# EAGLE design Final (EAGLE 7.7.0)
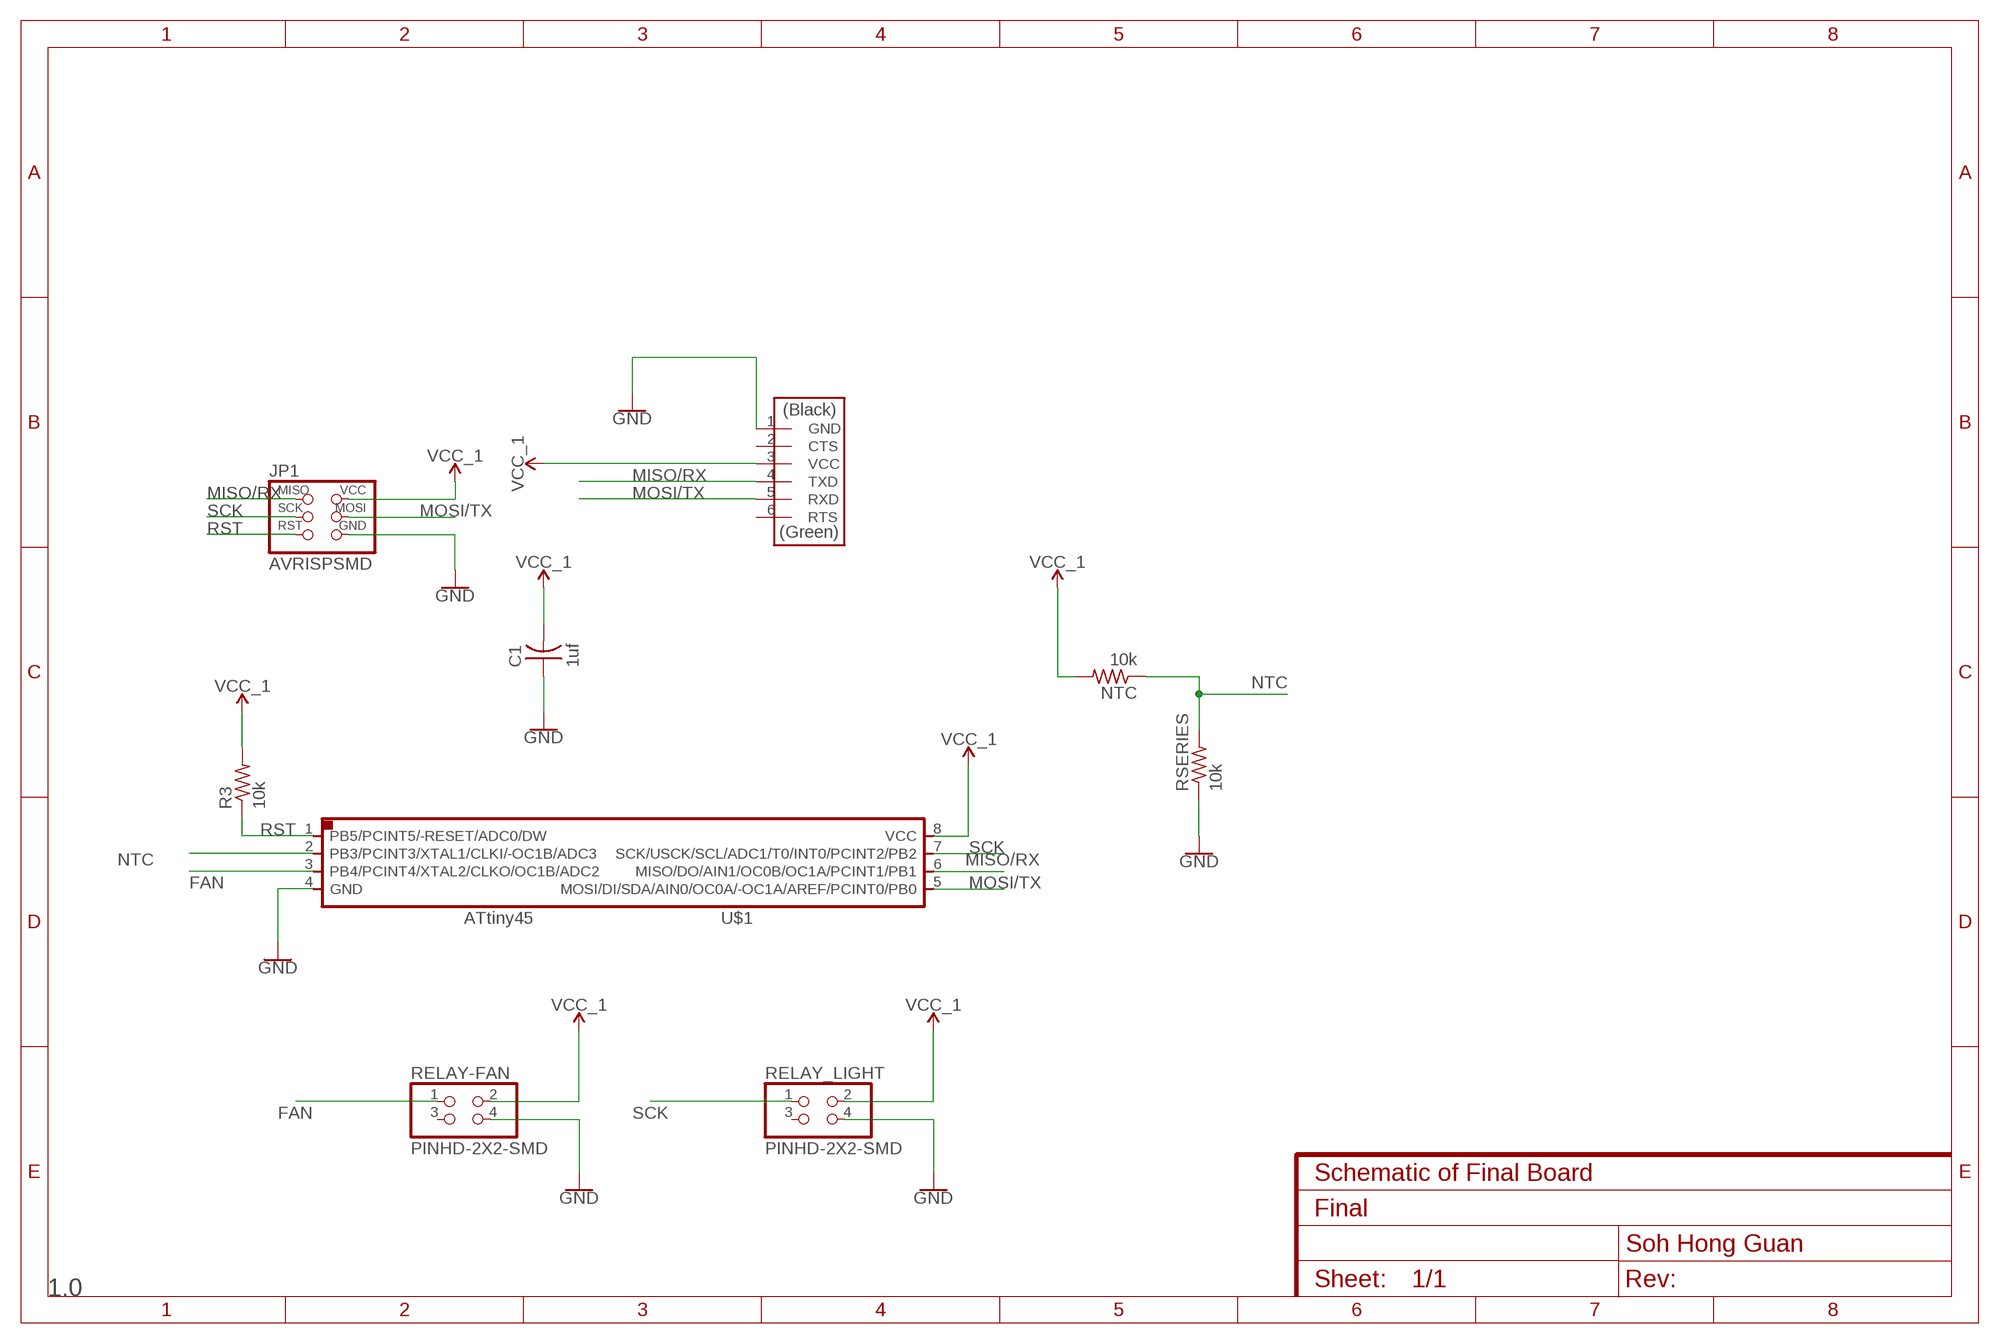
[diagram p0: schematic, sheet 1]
FRAME1 (FRAME-A4L): CNAME: Schematic of Final Board; CREVISION: 1.0; DESIGNER: Soh Hong Guan

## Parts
C1  1uf  CAP-US1206  [C1206]
JP1  AVRISPSMD  [2X03SMD]
NTC  10k  RES-US1206  [R1206]
R3  10k  RES-US1206  [R1206]
RELAY-FAN  PINHD-2X2-SMD  [2X02SMD]
RELAY_LIGHT  PINHD-2X2-SMD  [2X02SMD]
RSERIES  10k  RES-US1206  [R1206]
U$1  ATTINY45SI  [SOIC8]
U$3  FTDI-SMD-HEADER  [1X06SMD]

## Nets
FAN: RELAY-FAN.1 U$1.3(PB4/PCINT4/XTAL2/CLKO/OC1B/ADC2)
GND: C1.1 JP1.6(GND) RELAY-FAN.4 RELAY_LIGHT.4 RSERIES.1 U$1.4(GND) U$3.1(GND)
MISO/RX: JP1.1(MISO) U$1.6(MISO/DO/AIN1/OC0B/OC1A/PCINT1/PB1) U$3.4(TXD)
MOSI/TX: JP1.4(MOSI) U$1.5(MOSI/DI/SDA/AIN0/OC0A/-OC1A/AREF/PCINT0/PB0) U$3.5(RXD)
NTC: NTC.1 RSERIES.2 U$1.2(PB3/PCINT3/XTAL1/CLKI/-OC1B/ADC3)
RST: JP1.5(RST) R3.1 U$1.1(PB5/PCINT5/-RESET/ADC0/DW)
SCK: JP1.3(SCK) RELAY_LIGHT.1 U$1.7(SCK/USCK/SCL/ADC1/T0/INT0/PCINT2/PB2)
VCC_1: C1.2 JP1.2(VCC) NTC.2 R3.2 RELAY-FAN.2 RELAY_LIGHT.2 U$1.8(VCC) U$3.3(VCC)
Unconnected: RELAY-FAN.3 RELAY_LIGHT.3 U$3.2(CTS) U$3.6(RTS)

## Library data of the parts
C1 = fab:CAP-US
JP1 = fab:AVRISP
NTC R3 RSERIES = fab:RES-US: Resistor (US Symbol)
RELAY-FAN RELAY_LIGHT = fab:PINHD-2X2-SMD
U$1 = fab:ATTINY45
U$3 = fab:FTDI-SMD-HEADER

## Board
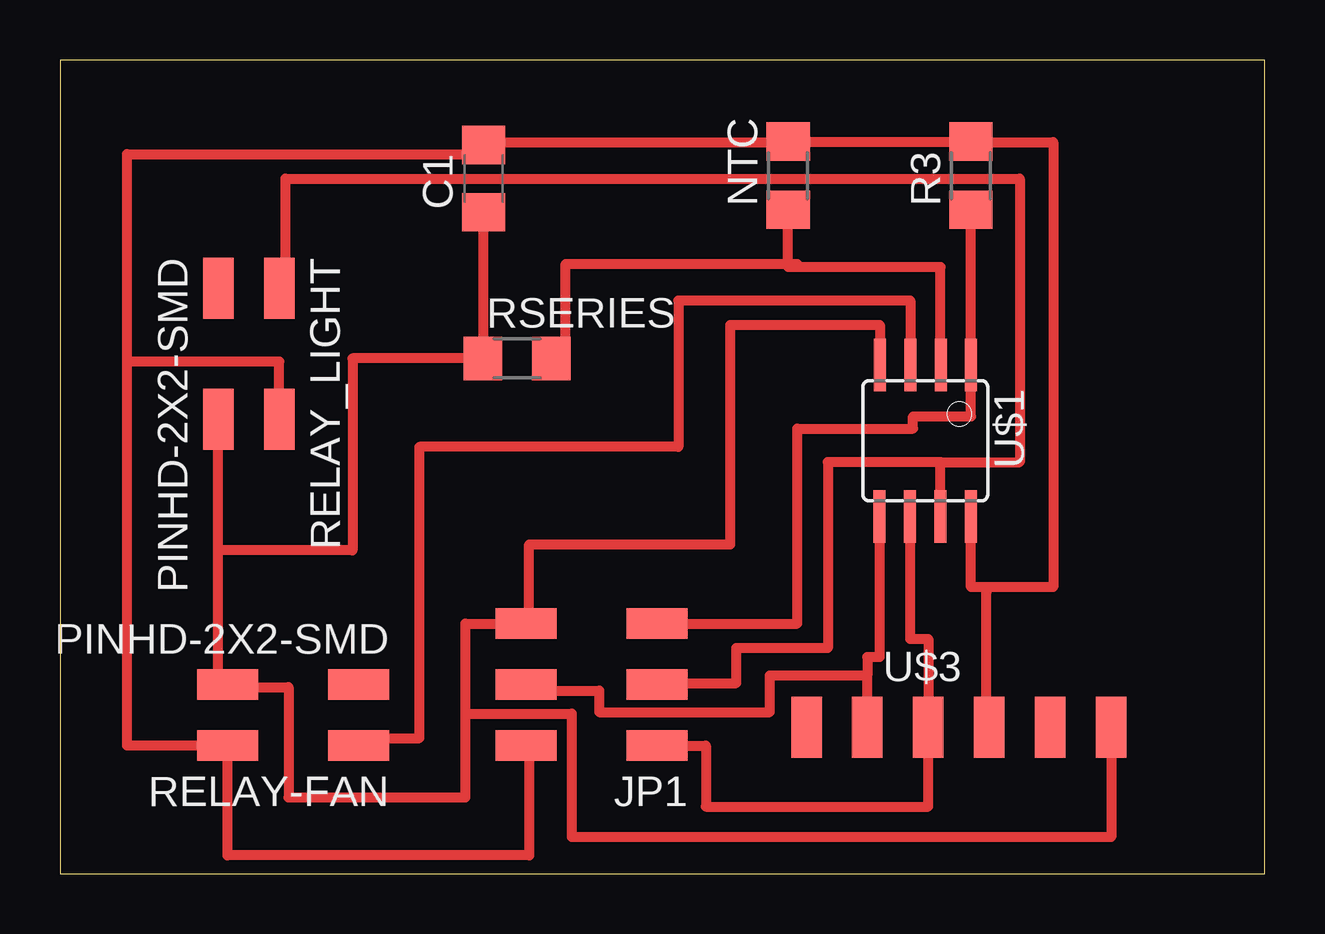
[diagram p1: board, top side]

Size 50.22 x 33.9 mm. Coordinates in mm from the lower left corner, seen from the top.
Outline: 0,0 50.22,0 50.22,33.9 0,33.9 0,0
Copper layers (1*16): Top 0.035mm / dielectric 1.5mm / Bottom 0.035mm
Design rules "default *": minimum track width 16mil, minimum drill 24mil, track to track 12mil, track to pad 12mil, pad to pad 12mil, via to via 8mil, smd to smd 12mil, copper to edge 40mil, drill to drill 8mil, minimum pad ring 10mil, minimum via ring 8mil, stop-mask expansion 4mil, vias tented up to drill 0mil, thermal gap 10mil

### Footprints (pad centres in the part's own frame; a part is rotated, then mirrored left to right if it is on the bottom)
C1206 = smd 1.6 x 1.8: 1 -1.4,0; 2 1.4,0
2X03SMD = smd 2.54 x 1.27: 1 -2.54,2.54; 2 2.92,2.54; 3 -2.54,0; 4 2.92,0; 5 -2.54,-2.54; 6 2.92,-2.54
R1206 = smd 1.6 x 1.803: 1 -1.422,0; 2 1.422,0
2X02SMD = smd 2.54 x 1.27: 1 -2.54,1.27; 2 2.92,1.27; 3 -2.54,-1.27; 4 2.92,-1.27
SOIC8 = smd 0.5 x 2.2: 1 -1.905,-3.154; 2 -0.645,-3.154; 3 0.625,-3.154; 4 1.895,-3.154; 5 1.905,3.154; 6 0.635,3.154; 7 -0.635,3.154; 8 -1.905,3.154
1X06SMD = smd 2.54 x 1.27: 1 0,6.35; 2 0,3.81; 3 0,1.27; 4 0,-1.27; 5 0,-3.81; 6 0,-6.35

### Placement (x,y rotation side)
C1  17.65,28.96 90 top
JP1  22.35,7.87 180 top
NTC  30.35,29.08 90 top
R3  37.97,29.08 90 top
RELAY-FAN  9.91,6.6 180 top
RELAY_LIGHT  7.87,21.84 270 top
RSERIES  19.05,21.46 0 top
U$1  36.07,18.03 180 top
U$3  37.47,6.1 270 top

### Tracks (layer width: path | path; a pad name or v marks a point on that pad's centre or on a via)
FAN
  Top 0.406: RELAY-FAN.1 12.45,5.64 14.99,5.64 14.99,17.78 25.78,17.78 25.78,23.88 35.44,23.88 U$1.3
GND
  Top 0.406: 34.14,20.93 U$1.4 34.17,22.86 27.94,22.86 27.94,13.72 19.56,13.72 19.56,10.62 JP1.6 | 19.2,10.62 JP1.6 | 6.6,19.15 6.76,19.15 RELAY_LIGHT.4 6.6,13.46 | JP1.6 16.89,10.41 16.89,6.67 | C1.1 17.63,27.56 RSERIES.1 12.19,21.46 12.19,13.46 6.6,13.46 | 6.6,13.46 6.6,8.13 7.11,8.13 RELAY-FAN.4 7.11,7.77 9.53,7.77 9.53,3.17 16.89,3.17 16.89,6.67 | 16.89,6.67 21.34,6.67 21.34,1.52 43.81,1.52 U$3.1
MISO/RX
  Top 0.406: JP1.1 26.92,5.33 26.92,2.79 36.2,2.79 U$3.4 36.2,9.78 35.43,9.78 U$1.6
MOSI/TX
  Top 0.406: U$3.5 33.66,8.26 | JP1.4 19.68,7.62 22.48,7.62 22.48,6.73 29.59,6.73 29.59,8.26 33.66,8.26 | U$1.5 34.16,9.02 33.66,9.02 33.66,8.26
NTC
  Top 0.406: U$1.2 36.7,25.27 30.73,25.27 | 30.73,25.27 30.35,25.27 NTC.1 | RSERIES.2 21.08,21.46 21.08,25.4 30.73,25.4 30.73,25.27
RST
  Top 0.406: JP1.5 30.73,10.41 30.73,18.54 35.56,18.54 35.56,19.05 37.97,19.05 U$1.1 R3.1
SCK
  Top 0.406: 9.25,24.49 RELAY_LIGHT.1 | 9.25,24.49 9.14,24.49 | U$1.7 36.7,17.14 | 36.7,17.14 40.01,17.14 40.01,28.96 9.4,28.96 9.4,24.49 9.25,24.49 | JP1.3 25.08,7.94 28.19,7.94 28.19,9.4 32,9.4 32,17.14 36.7,17.14
VCC_1
  Top 0.406: RELAY-FAN.2 7.11,5.28 6.99,5.28 | 19.56,5.28 JP1.2 19.2,5.28 19.56,5.28 | RELAY-FAN.2 6.99,0.76 19.56,0.76 19.56,5.28 | RELAY-FAN.2 2.79,5.33 2.79,21.34 | 2.79,21.34 2.79,29.97 17.65,29.97 C1.2 17.78,30.48 30.16,30.48 NTC.2 30.48,30.48 37.78,30.48 | RELAY_LIGHT.2 9.14,21.34 2.79,21.34 | 37.78,30.48 R3.2 | U$3.3 38.61,6.1 38.61,11.68 38.61,11.94 | 38.61,11.94 37.97,11.94 U$1.8 | 37.78,30.48 41.4,30.48 41.4,11.94 38.61,11.94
